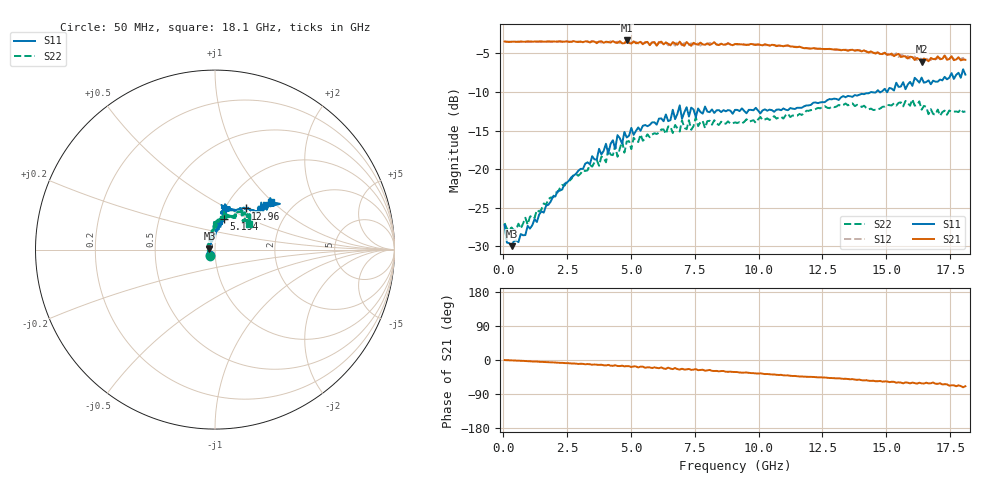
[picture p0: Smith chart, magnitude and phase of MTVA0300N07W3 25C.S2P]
! Network Analyzer HP8720D.06.14 Serial No. US36140669
!  7 Jul 2005  11:41:23
! Frequency  S11  S21  S12  S22
# HZ  S  DB R 50
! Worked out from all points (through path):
!   201 points, 50 MHz to 18.1 GHz, reference 50 ohm
!   highest |S21| = -3.33 dB at 4.833 GHz (marker M1); lowest = -6.1 dB at 16.39 GHz (marker M2)
!   group delay of S21, straight-line fit = 10.7 ps
!   lowest |S11| = -30.0 dB at 320.8 MHz (marker M3), VSWR 1.07, Z = 47 + j0.475 ohm
!   |S11| at or under -10 dB: start of sweep to 14.6 GHz; 14.74038 GHz to 14.79263 GHz (52.25 MHz wide, 0.354 % of centre); 15.0234 GHz to 15.03803 GHz (14.63 MHz wide, 0.0974 % of centre)
!   |S22| runs from -27.9 to -11.0 dB; largest |S21 - S12| = 0.038
!   S11 on the Smith chart (normalised r, x): 50 MHz: 0.94, -0.06; 5.194 GHz: 1.04, +0.36; 12.96 GHz: 1.24, +0.62; 18.1 GHz: 1.53, +0.97
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5e7  -27.22 -133.9  -3.47 -0.2  -3.48 -0.3  -26.99 -124.5
1.4025e8  -29.51 -164.4  -3.50 -0.5  -3.50 -0.5  -27.71 -164.4
3.2075e8  -29.98 170.8  -3.50 -0.9  -3.51 -1.0  -27.56 173.9
9.525e8  -27.34 127.6  -3.46 -2.9  -3.49 -2.9  -27.19 141.5
3.1185e9  -19.98 86.4  -3.55 -10.1  -3.56 -10.7  -20.16 102.0
4.47225e9  -15.60 74.9  -3.66 -15.8  -3.50 -14.4  -18.39 95.5
4.65275e9  -16.72 75.0  -3.71 -15.0  -3.47 -16.4  -16.38 93.7
4.743e9  -15.19 77.8  -3.69 -16.8  -3.64 -15.5  -17.87 89.7
4.83325e9  -15.90 83.0  -3.33 -16.2  -3.57 -17.5  -16.42 82.9
5.19425e9  -15.05 73.6  -3.70 -16.9  -3.51 -17.1  -16.33 91.3
6.09675e9  -13.46 75.1  -3.60 -21.7  -3.52 -21.3  -15.27 80.3
6.7285e9  -13.52 81.1  -3.72 -21.2  -4.00 -22.6  -14.28 73.6
6.909e9  -11.74 77.6  -3.49 -25.2  -3.66 -23.2  -15.13 73.4
6.99925e9  -13.47 77.5  -3.84 -23.2  -3.96 -25.6  -13.67 73.7
7.17975e9  -11.99 81.8  -3.53 -24.8  -3.88 -23.7  -14.83 69.2
7.54075e9  -13.26 73.6  -3.81 -24.1  -3.61 -27.1  -13.29 76.5
9.075e9  -12.32 74.7  -3.80 -31.6  -3.77 -31.7  -13.95 66.0
1.21435e10  -11.39 58.8  -4.33 -44.7  -4.29 -44.8  -12.31 59.0
1.295575e10  -10.87 53.4  -4.52 -48.0  -4.47 -48.1  -11.98 56.5
1.512175e10  -9.49 40.2  -5.17 -58.5  -4.93 -57.8  -11.72 51.3
1.638525e10  -8.14 39.3  -6.07 -61.6  -5.72 -60.4  -12.30 42.4
1.81e10  -7.76 40.4  -5.84 -69.2  -6.14 -70.0  -12.53 37.1
